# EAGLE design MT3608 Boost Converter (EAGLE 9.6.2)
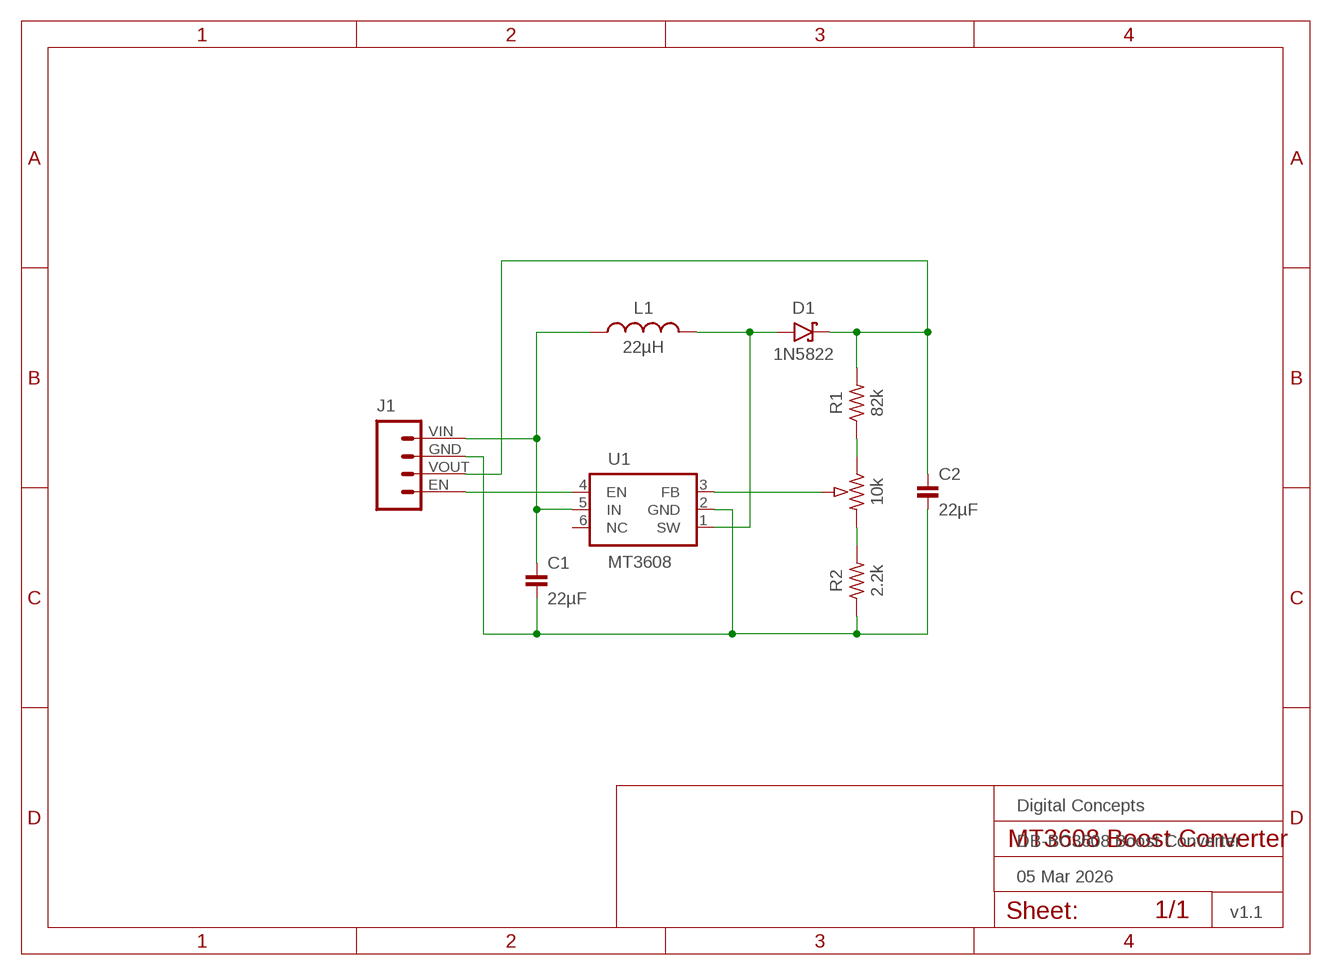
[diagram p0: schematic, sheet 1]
FRAME2 (FRAME_A5L-LOC): DATE: 05 Mar 2026; OWNER: Digital Concepts; TITLE: DB-BC3608 Boost Converter; VERSION: v1.1

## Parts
C1  22µF  CAPACITOR-0805  [C0805]
C2  22µF  CAPACITOR-0805  [C0805]
D1  1N5822  DIODE-SCHOTTKY-1N5822  [DIODE_SMB]
J1  HEADER-1X4-BOOST  [CONN_04-BOOST]
L1  22µH  INDUCTOR-CDRH104R/6D28L5038P  [CDRH104R+6D28]
R1  82k  RESISTOR-0603  [R0603]
R2  2.2k  RESISTOR-0603  [R0603]
U1  MT3608  [SOT-23-6]
VOUT  10k  RESISTOR-TRIMM-33-US  [RTRIM3*3]

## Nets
EN: J1.EN U1.4(EN)
GND: C1.2 C2.2 J1.GND R2.1 U1.2(GND)
N$1: D1.A L1.1 U1.1(SW)
N$2: U1.3(FB) VOUT.2(S)
N$3: R1.1 VOUT.1(A)
N$4: R2.2 VOUT.3(E)
VIN: C1.1 J1.VIN L1.2 U1.5(IN)
VOUT: C2.1 D1.C J1.VOUT R1.2
Unconnected: U1.6(NC)

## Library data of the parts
C1 C2 = digitalconcepts:CAPACITOR-0805: 0805 Capacitor
D1 = digitalconcepts:DIODE-SCHOTTKY-1N5822: 1N5822 Schottky Diode SMB
J1 = digitalconcepts:HEADER-1X4-BOOST: Boost Converter Module 4-Pin Header
L1 = digitalconcepts:INDUCTOR-CDRH104R/6D28: Inductor; SPICEPREFIX: L
R1 R2 = digitalconcepts:RESISTOR-0603: Resistor
U1 = digitalconcepts:MT3608: MT3608 DC-DC Step-Up Voltage Converter
VOUT = digitalconcepts:RESISTOR-TRIMM-3*3-US: Trimm Resistor - 3*3 SMD

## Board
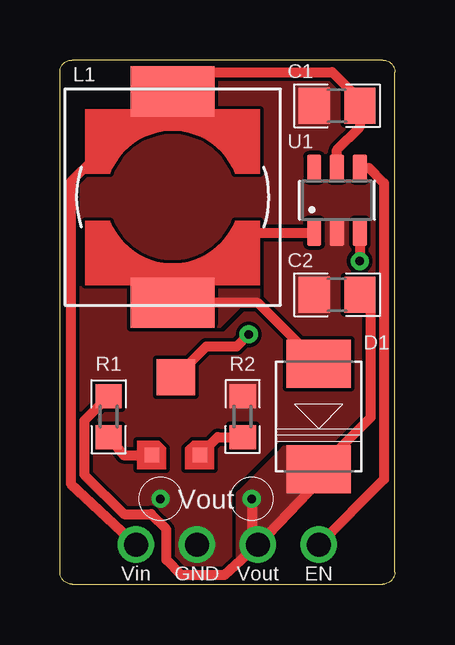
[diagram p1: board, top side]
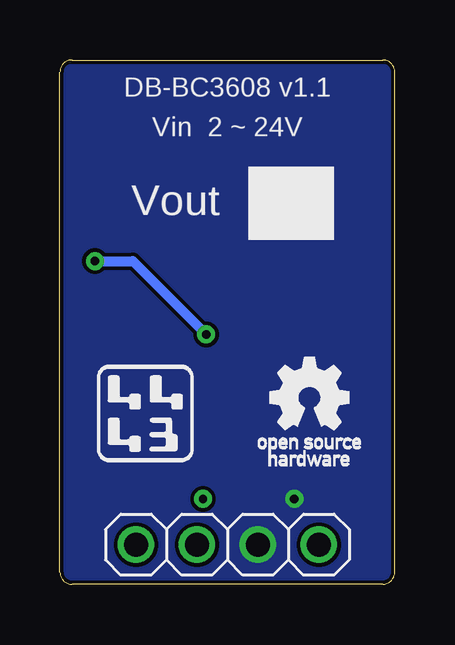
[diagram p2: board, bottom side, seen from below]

Size 13.97 x 21.84 mm. Coordinates in mm from the lower left corner, seen from the top.
Outline: 0.51,0 arc-90 0,0.51 0,21.34 arc-90 0.51,21.84 13.46,21.84 arc-90 13.97,21.34 13.97,0.51 arc-90 13.46,0 0.51,0
Copper layers (1*16): Top 0.035mm / dielectric 1.5mm / Bottom 0.035mm
Design rules "default *": minimum track width 6mil, minimum drill 0.15mm, track to track 6mil, track to pad 6mil, pad to pad 6mil, via to via 6mil, smd to smd 6mil, copper to edge 6mil, drill to drill 6mil, minimum pad ring 10mil, minimum via ring 8mil, stop-mask expansion 4mil, vias tented up to drill 0mil, thermal gap 0mil

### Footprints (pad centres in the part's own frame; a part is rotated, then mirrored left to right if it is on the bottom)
C0805 = smd 1.3 x 1.5: 1 -0.95,0; 2 0.95,0
DIODE_SMB = smd 2 x 2.7: A 2.2,0; C -2.2,0
CONN_04-BOOST = drill 1 pad 1.524: EN 0,0; GND 5.08,0; VIN 7.62,0; VOUT 2.54,0
CDRH104R+6D28 = smd 2.1 x 3.5: 1 -4.4,0; 2 4.4,0
R0603 = smd 1 x 1.1: 1 -0.85,0; 2 0.85,0
SOT-23-6 = smd 1.1 x 0.6: 1 -1.35,0.95; 2 -1.35,0; 3 -1.35,-0.95; 4 1.35,-0.95; 5 1.35,0; 6 1.35,0.95
RTRIM3*3 = smd 0.6 x 0.6: 1 -1,-1.6; 3 1,-1.6 | smd 1.6 x 1.5: 2 0,1.65

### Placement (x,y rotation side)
C1  11.56,19.94 180 top
C2  11.56,12.06 180 top
D1  10.79,6.99 90 top
J1  10.79,1.65 0 bottom
L1  4.7,16.13 90 top
R1  2.03,6.99 90 top
R2  7.62,6.99 270 top
U1  11.56,16 90 top
VOUT  4.83,6.99 0 top

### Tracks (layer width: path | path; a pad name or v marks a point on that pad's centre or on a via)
EN
  Top 0.406: J1.EN 13.51,4.37 13.51,16.72 12.89,17.35 U1.4
GND  (via drill 0.35)
  other vias: 4.19,3.56
  pour Top (rank 5): 14.86,22.48 14.86,-0.76 -0.89,-0.76 -0.89,22.48
  pour Bottom: 14.48,22.23 14.48,-0.51 -0.51,-0.51 -0.51,22.23
N$1
  Top 0.406: D1.A 8.26,11.72 L1.1 7.45,14.65 U1.1
  pour Top (no thermals): 6.35,10.74 6.68,10.74 7.52,11.58 8.28,11.58 8.28,12.57 6.35,12.57
N$2  (via drill 0.35)
  Top 0.406: VOUT.2 6.1,9.9 7.37,9.9 v7.87,10.41 | U1.3 v12.51,13.46
  Bottom 0.406: v12.51,13.46 10.92,13.46 v7.87,10.41
N$3
  Top 0.406: R1.1 2.65,5.38 VOUT.1
N$4
  Top 0.406: VOUT.3 6.58,6.13 R2.2
VIN
  Top 0.406: U1.5 11.56,18.1 12.51,19.05 C1.1 12.76,19.94 11.36,21.34 5.51,21.34 L1.2 4.27,20.53 0.46,16.76 0.46,4.19 J1.VIN
VOUT  (via drill 0.35)
  Top 0.406: C2.1 12.95,11.62 12.95,6.94 D1.C 10.79,4.31 J1.VOUT | R1.2 1.02,6.82 1.02,4.57 2.67,2.92 3.81,2.92 4.45,2.29 4.45,1.02 5.08,0.38 6.86,0.38 J1.VOUT | v8,3.56 8,1.91 J1.VOUT
  pour Top (no thermals): 7.54,1.02 7.54,3.73 9.4,5.59 10.41,5.59 10.41,3.89

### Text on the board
bPlace: DB-BC3608 v1.1 | Vin 2 ~ 24V | Vout
tNames: Vout | Vin | GND | Vout | EN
